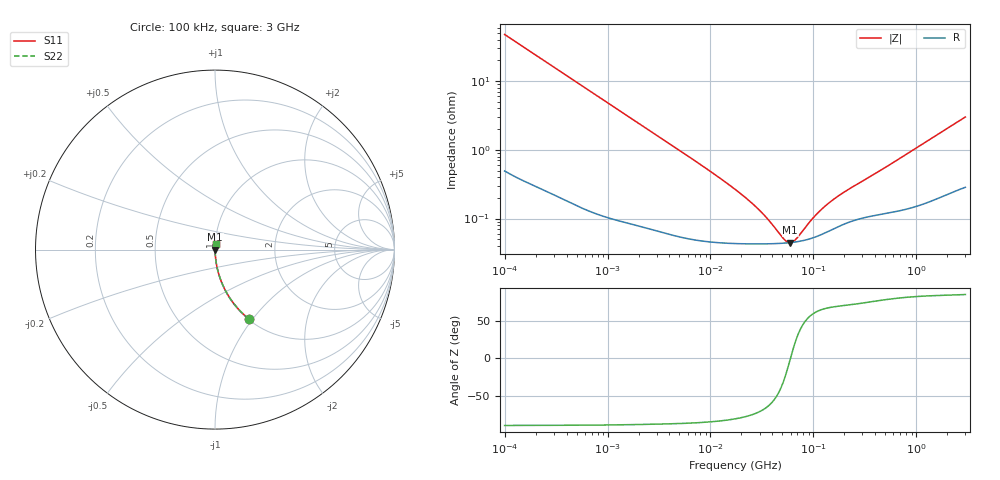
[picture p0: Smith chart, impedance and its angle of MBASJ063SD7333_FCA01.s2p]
! MBASJ063SD7333_FCA01  S-PARAMETER MODEL  ( Standard Model )
! Model Generated by TAIYO YUDEN Corporation (http://www.ty-top.com)
! Version 1.0
! TAIYO YUDEN Control No. 220601
! Copyright(c) 2022 TAIYO YUDEN CO.,LTD. All Rights Reserved.
! Product Description (link to TY-COMPAS)
! https://ds.yuden.co.jp/TYCOMPAS/or/detail?pn=MBASJ063SD7333KFCA01&u=M
! Products Name : Multilayer Ceramic Capacitors
! Characteristics :
!  Capacitance : 0.033 [uF] , Rated Voltage : 6.3 [V] , TCC : X7T
!  Case Size : 0.6 x 0.3 / 0.024 x 0.012 [mm/inch] , Thickness : 0.3 / 0.012 [mm/inch]
!  (Conditions: Temperature = 25 [degC] , DC Bias Voltage = 0 [V])
! External Node Assignments :
!  1  o---| |---o  2
! GND o---------o GND
! Frequency Range : 100kHz  -  3GHz  [ 401 STEP ]
# MHZ S RI R 50
! Freq[MHz].  S11 Real  S11 Imag  S21 Real  S21 Imag  S12 Real  S12 Imag  S22 Real  S22 Imag
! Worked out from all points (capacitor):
!   401 points, 100 kHz to 3 GHz, reference 50 ohm
!   read as one part in series: C = 33.2 nF near 105.3 kHz
!   lowest |Z| = 44.7 mohm at 59.68 MHz (marker M1)
!   series resonance near 59.95 MHz, so ESL is about 210 pH
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0.1  0.1886 -0.3861  0.8114 0.3861  0.8114 0.3861  0.1886 -0.3861
0.14345  0.103 -0.2984  0.897 0.2984  0.897 0.2984  0.103 -0.2984
0.200542  0.0566 -0.2251  0.9434 0.2251  0.9434 0.2251  0.0566 -0.2251
0.327242  0.0232 -0.1435  0.9768 0.1435  0.9768 0.1435  0.0232 -0.1435
0.562235  0.00873 -0.0851  0.9913 0.0851  0.9913 0.0851  0.00873 -0.0851
1.18716  0.00262 -0.0408  0.9974 0.0408  0.9974 0.0408  0.00262 -0.0408
3.161081  0.000886 -0.0155  0.9991 0.0155  0.9991 0.0155  0.000886 -0.0155
9.093698  0.000491 -0.00533  0.9995 0.00533  0.9995 0.00533  0.000491 -0.00533
17.7727  0.000438 -0.00255  0.9996 0.00255  0.9996 0.00255  0.000438 -0.00255
24.21403  0.000431 -0.00172  0.9996 0.00172  0.9996 0.00172  0.000431 -0.00172
31.3325  0.000429 -0.00116  0.9996 0.00116  0.9996 0.00116  0.000429 -0.00116
37.52708  0.00043 -0.000809  0.9996 0.000809  0.9996 0.000809  0.00043 -0.000809
52.46276  0.000439 -0.000223  0.9996 0.000223  0.9996 0.000223  0.000439 -0.000223
56.67997  0.000443 -9.35e-05  0.9996 9.35e-05  0.9996 9.35e-05  0.000443 -9.35e-05
59.67813  0.000446 -7.39e-06  0.9996 7.39e-06  0.9996 7.39e-06  0.000446 -7.39e-06
62.83488  0.00045 7.88e-05  0.9995 -7.88e-05  0.9995 -7.88e-05  0.00045 7.88e-05
67.88584  0.000458 0.000208  0.9995 -0.000208  0.9995 -0.000208  0.000458 0.000208
97.38194  0.00052 0.000837  0.9995 -0.000837  0.9995 -0.000837  0.00052 0.000837
126.0104  0.000607 0.00132  0.9994 -0.00132  0.9994 -0.00132  0.000607 0.00132
171.6802  0.000756 0.00195  0.9992 -0.00195  0.9992 -0.00195  0.000756 0.00195
547.5153  0.00124 0.0059  0.9988 -0.0059  0.9988 -0.0059  0.00124 0.0059
3000  0.00373 0.0298  0.9963 -0.0298  0.9963 -0.0298  0.00373 0.0298
